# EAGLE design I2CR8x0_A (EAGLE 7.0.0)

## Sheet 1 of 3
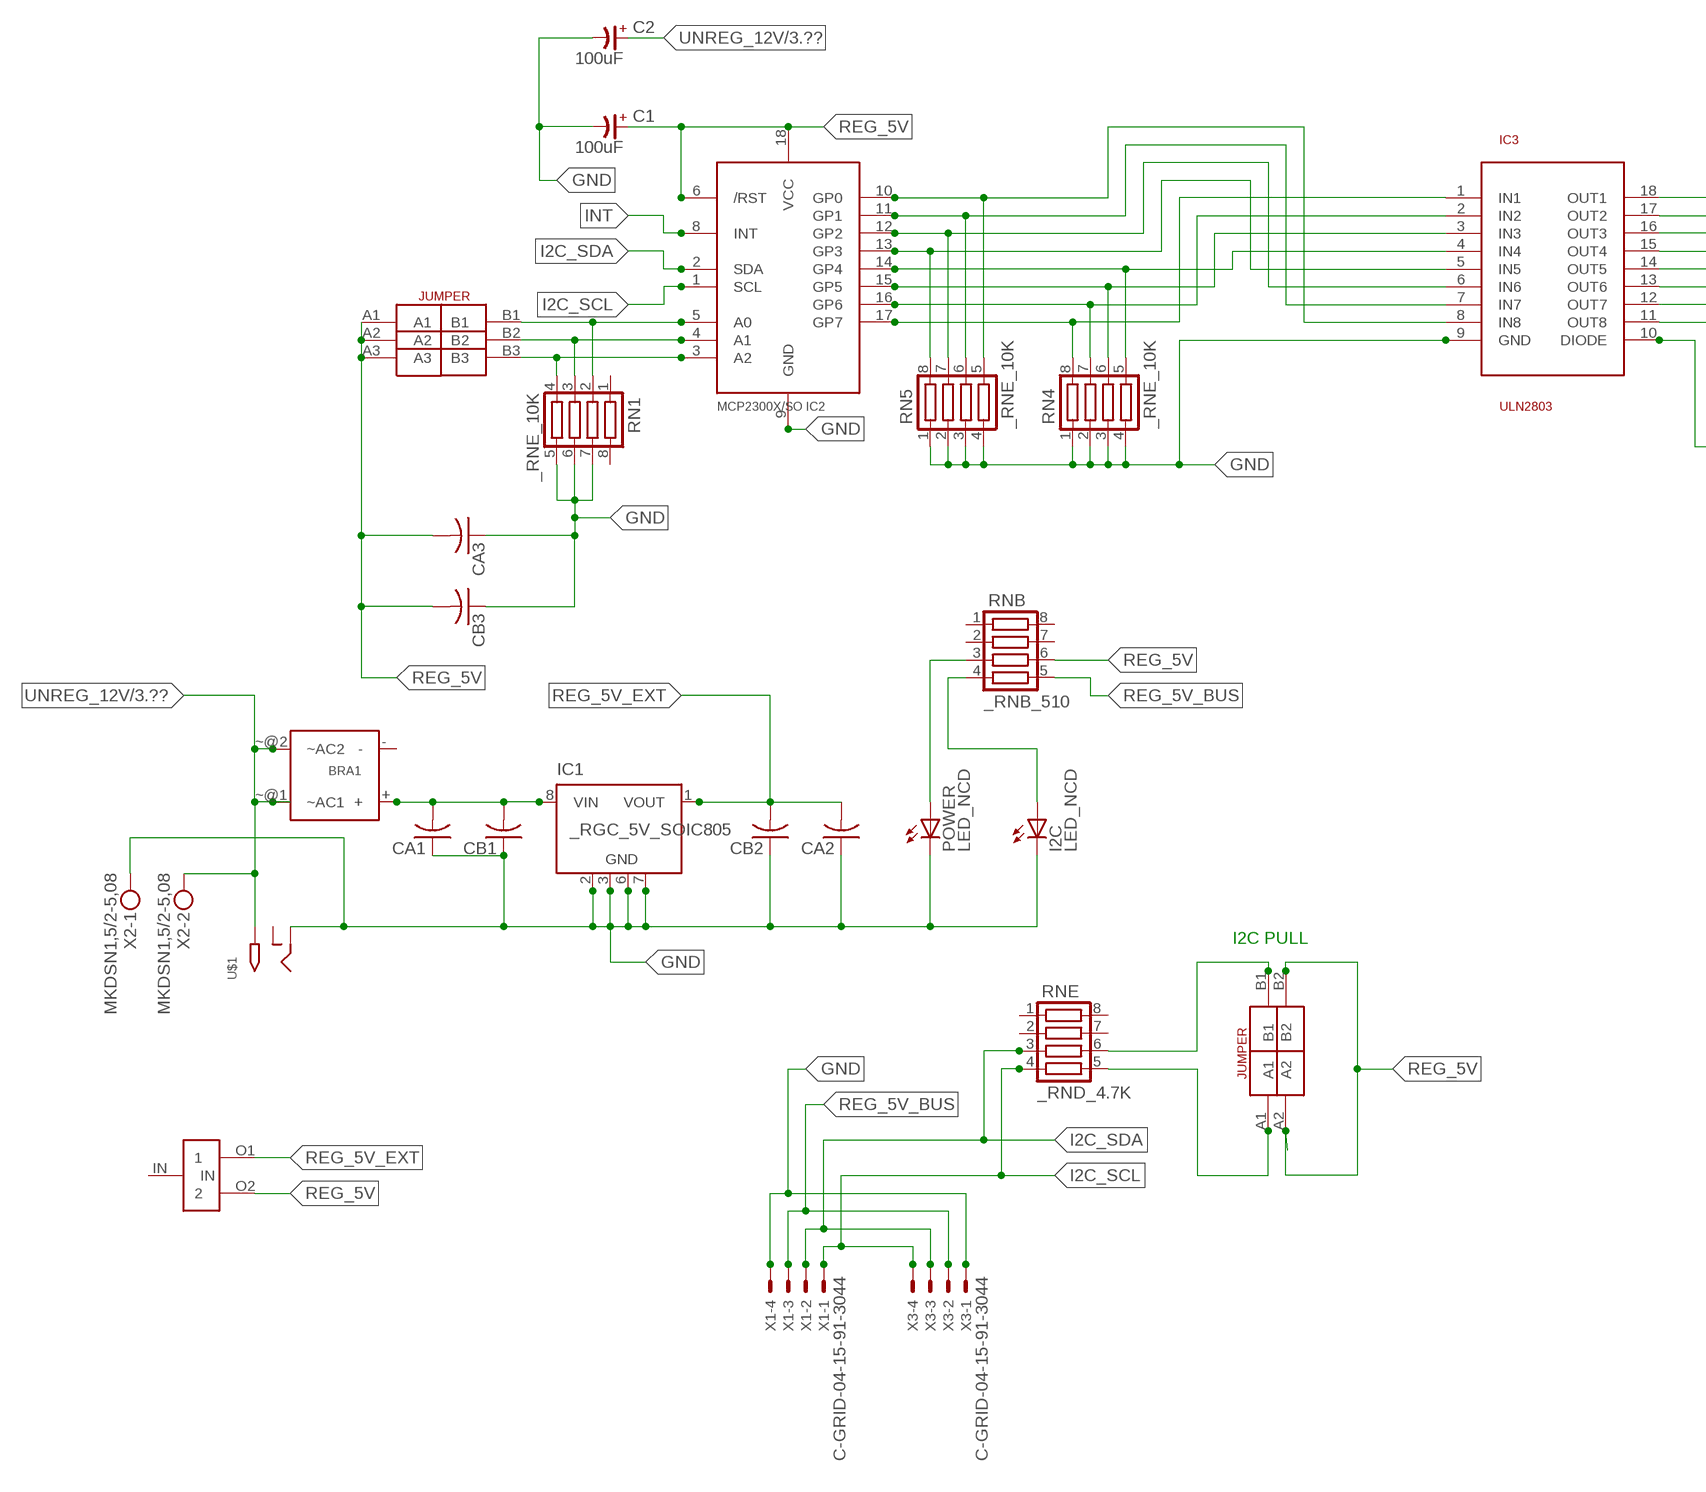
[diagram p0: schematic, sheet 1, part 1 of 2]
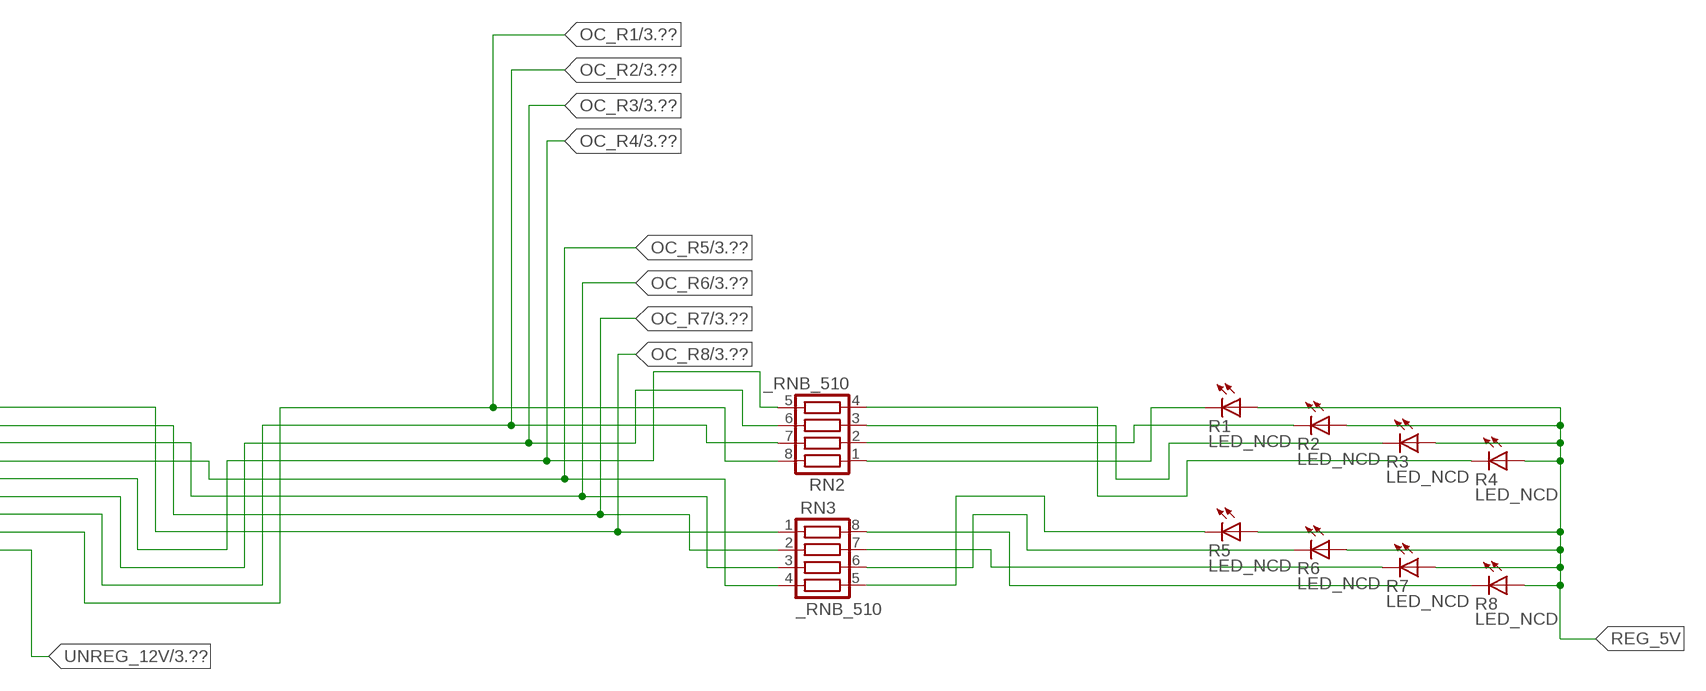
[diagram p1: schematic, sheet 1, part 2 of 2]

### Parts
BRA1  MB2S_  [MB2S]
C1  100uF  CP-E-025X060  [E-025X060]
C2  100uF  CP-E-025X060  [E-025X060]
CA1  CC1206KRX7R9BB104C1206K  [CC1206KRX7R9BB104]
CA2  CC1206KRX7R9BB104C1206K  [CC1206KRX7R9BB104]
CA3  CC1206KRX7R9BB104C1206K  [CC1206KRX7R9BB104]
CB1  TMK316F106ZL-TC1206K  [TMK316F106ZL-T]
CB2  TMK316F106ZL-TC1206K  [TMK316F106ZL-T]
CB3  TMK316F106ZL-TC1206K  [TMK316F106ZL-T]
I2C  LED_NCD  [CHIPLED_0603]
IC1  _RGC_5V_SOIC805  [_RGC_5V_SOIC8]
IC2  MCP2300X/SO  [SO18W]
IC3  ULN2803  [SO18L]
POWER  LED_NCD  [CHIPLED_0603]
R1  LED_NCD  [CHIPLED_0603]
R2  LED_NCD  [CHIPLED_0603]
R3  LED_NCD  [CHIPLED_0603]
R4  LED_NCD  [CHIPLED_0603]
R5  LED_NCD  [CHIPLED_0603]
R6  LED_NCD  [CHIPLED_0603]
R7  LED_NCD  [CHIPLED_0603]
R8  LED_NCD  [CHIPLED_0603]
RN1  _RNE_10K  [RNE]
RN2  _RNB_510  [RNB]
RN3  _RNB_510  [RNB]
RN4  _RNE_10K  [RNE]
RN5  _RNE_10K  [RNE]
RNB  _RNB_510  [RNB]
RNE  _RND_4.7K  [RND]
U$1  2.1MMJACK  [PJ-102A]
U$3  JUMPER_2X2  [JUMPER_2X2]
U$5  LINK_2  [LINK_2]
U$18  JUMPER_3X2  [JUMPER_3X2]
X1  C-GRID-04-15-91-3044  [15-91-04]
X2  MKDSN1,5/2-5,08  [MKDSN1,5/2-5,08]
X3  C-GRID-04-15-91-3044  [15-91-04]

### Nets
GND: C1.- C2.- CA1.1 CA2.1 CA3.1 CB1.1 CB2.1 CB3.1 I2C.C IC1.2(GND) IC1.3(GND) IC1.6(GND) IC1.7(GND) IC2.9(GND) IC3.9(GND) POWER.C RN1.5 RN1.6 RN1.7 RN4.1 RN4.2 RN4.3 RN4.4 RN5.1 RN5.2 RN5.3 RN5.4 U$1.RING X1.4 X2.1 X3.1
GP4: IC2.14(GP4) IC3.4(IN4) RN4.5
GP6: IC2.16(GP6) IC3.2(IN2) RN4.7
I2C_SCL: IC2.1(SCL) RNE.4 X1.1 X3.4
I2C_SDA: IC2.2(SDA) RNE.3 X1.2 X3.3
INT: IC2.8(INT)
N$1: BRA1.+ CA1.2 CB1.2 IC1.8(VIN)
N$2: POWER.A RNB.3
N$3: I2C.A RNB.4
N$4: RNE.5 U$3.A1
N$5: RNE.6 U$3.B1
N$6: IC2.5(A0) RN1.2 U$18.B1
N$7: IC2.4(A1) RN1.3 U$18.B2
N$8: IC2.3(A2) RN1.4 U$18.B3
N$20: R1.C RN2.1
N$21: IC2.12(GP2) IC3.6(IN6) RN5.7
N$22: IC2.11(GP1) IC3.7(IN7) RN5.6
N$23: IC2.10(GP0) IC3.8(IN8) RN5.5
N$29: R2.C RN2.2
N$30: R3.C RN2.3
N$31: R4.C RN2.4
N$32: R8.C RN3.8
N$81: R7.C RN3.7
N$82: R6.C RN3.6
N$83: R5.C RN3.5
N$89: IC2.13(GP3) IC3.5(IN5) RN5.8
N$93: IC2.15(GP5) IC3.3(IN3) RN4.6
N$94: IC2.17(GP7) IC3.1(IN1) RN4.8
OC_R1: IC3.11(OUT8) RN2.8 ; also sheet 3
OC_R2: IC3.12(OUT7) RN2.7 ; also sheet 3
OC_R3: IC3.13(OUT6) RN2.6 ; also sheet 3
OC_R4: IC3.14(OUT5) RN2.5 ; also sheet 3
OC_R5: IC3.15(OUT4) RN3.4 ; also sheet 3
OC_R6: IC3.16(OUT3) RN3.3 ; also sheet 3
OC_R7: IC3.17(OUT2) RN3.2 ; also sheet 3
OC_R8: IC3.18(OUT1) RN3.1 ; also sheet 3
REG_5V: C1.+ CA3.2 CB3.2 IC2.6(/RST) IC2.18(VCC) R1.A R2.A R3.A R4.A R5.A R6.A R7.A R8.A RNB.6 U$3.A2 U$3.B2 U$5.O2 U$18.A1 U$18.A2 U$18.A3
REG_5V_BUS: RNB.5 X1.3 X3.2
REG_5V_EXT: CA2.2 CB2.2 IC1.1(VOUT) U$5.O1
UNREG_12V: BRA1.~@1(~AC1) BRA1.~@2(~AC2) C2.+ IC3.10(DIODE) U$1.TIP X2.2 ; also sheet 3
Unconnected: BRA1.- IC1.4(NC) IC1.5(NC) RN1.1 RN1.8 RNB.1 RNB.2 RNB.7 RNB.8 RNE.1 RNE.2 RNE.7 RNE.8 U$1.RING_SW U$5.IN

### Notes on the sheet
- I2C PULL

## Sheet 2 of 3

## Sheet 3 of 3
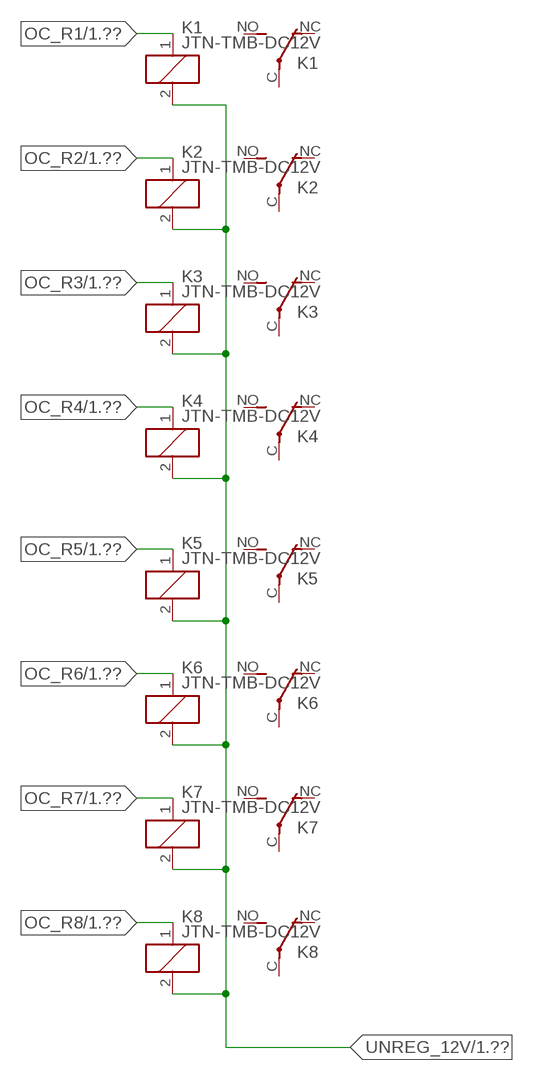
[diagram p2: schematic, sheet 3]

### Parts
K1  JTN-TMB-DC12V  [JT-TMB]
K2  JTN-TMB-DC12V  [JT-TMB]
K3  JTN-TMB-DC12V  [JT-TMB]
K4  JTN-TMB-DC12V  [JT-TMB]
K5  JTN-TMB-DC12V  [JT-TMB]
K6  JTN-TMB-DC12V  [JT-TMB]
K7  JTN-TMB-DC12V  [JT-TMB]
K8  JTN-TMB-DC12V  [JT-TMB]

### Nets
OC_R1: K1.1(C1) ; also sheet 1
OC_R2: K2.1(C1) ; also sheet 1
OC_R3: K3.1(C1) ; also sheet 1
OC_R4: K4.1(C1) ; also sheet 1
OC_R5: K5.1(C1) ; also sheet 1
OC_R6: K6.1(C1) ; also sheet 1
OC_R7: K7.1(C1) ; also sheet 1
OC_R8: K8.1(C1) ; also sheet 1
UNREG_12V: K1.2(C2) K2.2(C2) K3.2(C2) K4.2(C2) K5.2(C2) K6.2(C2) K7.2(C2) K8.2(C2) ; also sheet 1
Unconnected: K1.C(COM) K1.NC K1.NO K2.C(COM) K2.NC K2.NO K3.C(COM) K3.NC K3.NO K4.C(COM) K4.NC K4.NO K5.C(COM) K5.NC K5.NO K6.C(COM) K6.NC K6.NO K7.C(COM) K7.NC K7.NO K8.C(COM) K8.NC K8.NO

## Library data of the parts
BRA1 = NCD_ULTIMATE_LIBRARY:MB2S: Bridge Rectifier BRA MB2S 200V 500ma Digikey MB2S-TPMSTR-ND/MB2S-TP
C1 C2 = NCD_ULTIMATE_LIBRARY:CP-: Capacitors All Kinds POLARIZED CAP
CA1-CA3 = NCD_ULTIMATE_LIBRARY:CC1206KRX7R9BB104: Capacitor CA .1uF 50V SMT C1206K CC1206KRX7R9BB104
CB1-CB3 = NCD_ULTIMATE_LIBRARY:TMK316F106ZL-T: Capacitor CB 10uF SMT 1206 TMK316F106ZL-T
I2C POWER = NCD_ULTIMATE_bhaskar:LED_NCD
IC1 = NCD_ULTIMATE_LIBRARY:_RGC_5V_SOIC8: Regulator Linear 5V Chip Positive VOLTAGE REGULATOR Digikey 497-7267-2-ND/L78L05CD13TR
IC2 = NCD_ULTIMATE_LIBRARY:MCP2300X: Semiconductor Port Expander I/O 8-Bit I2C MCP23008 Inexpensive i2c i/o expander - 8 general purpose i/o pins with optional pullups
IC3 = NCD_ULTIMATE_LIBRARY:ULN2803: Semiconductor 8 O.C. N-Channel Transistor Driver Digikey ULN2803AFWGCELTR-ND/ULN2803AFWG,C,EL
K1-K8 = NCD_ULTIMATE_LIBRARY:JT?-*: RELAY COMPACT ECONOMICAL 30 AMP. RELAY NAiS Source: http://www.mew-europe.com/.. en_ds_61212_0000.pdf
R1-R8 = NCD_ULTIMATE_LIBRARY:LED_NCD: LED Digikey 754-1132-2-ND/APT2012SRCPRV
RN1 RN4 RN5 = NCD_ULTIMATE_LIBRARY:_RNE_10K: Resistor Array RNE SMT 10K x 4 Single Resistor Source: http://www.ctscorp.com/components/Datasheets/CTSChipArrayDs.pdf Digikey 742C083103JPTR-ND/742C083103JP; OC_FARNELL: unknown; OC_NEWARK: unknown
RN2 RN3 RNB = NCD_ULTIMATE_LIBRARY:_RNB_510: Resistor Array RNB SMT 510 x 4 Single Resistor Source: http://www.ctscorp.com/components/Datasheets/CTSChipArrayDs.pdf Digikey 742C083511JPTR-ND/ 742C083511JP; OC_FARNELL: unknown; OC_NEWARK: unknown
RNE = NCD_ULTIMATE_LIBRARY:_RND_4.7K: Resistor Array RND SMT 4.7K x 4 Single Resistor Source: http://www.ctscorp.com/components/Datasheets/CTSChipArrayDs.pdf Digikey 742C083472JPTR-ND/742C083472JP; OC_FARNELL: unknown; OC_NEWARK: unknown
U$1 = NCD_ULTIMATE_CONNECTORS:2.1MMJACK: 2.1mm x 5.5mm DC jack with internal switch. Digikey part #PJ-102A, 4UCON part #05537 By microbuilder.eu
U$3 = NCD_ULTIMATE_CONNECTORS:JUMPER_2X2
U$5 = NCD_ULTIMATE_LIBRARY:LINK_2: PAD_top
U$18 = NCD_ULTIMATE_CONNECTORS:JUMPER_3X2
X1 X3 = NCD_ULTIMATE_CONNECTORS:C-GRID-04: CONNECTOR 4-Pos I2C wire to board 2.54 mm (0.100") pitch header Digikey WM1342-ND/0015912045; OC_FARNELL: unknown; OC_NEWARK: unknown
X2 = NCD_ULTIMATE_CONNECTORS:MKDSN1,5/2-5,08: MKDSN 1,5/ 2-5,08 Printklemme

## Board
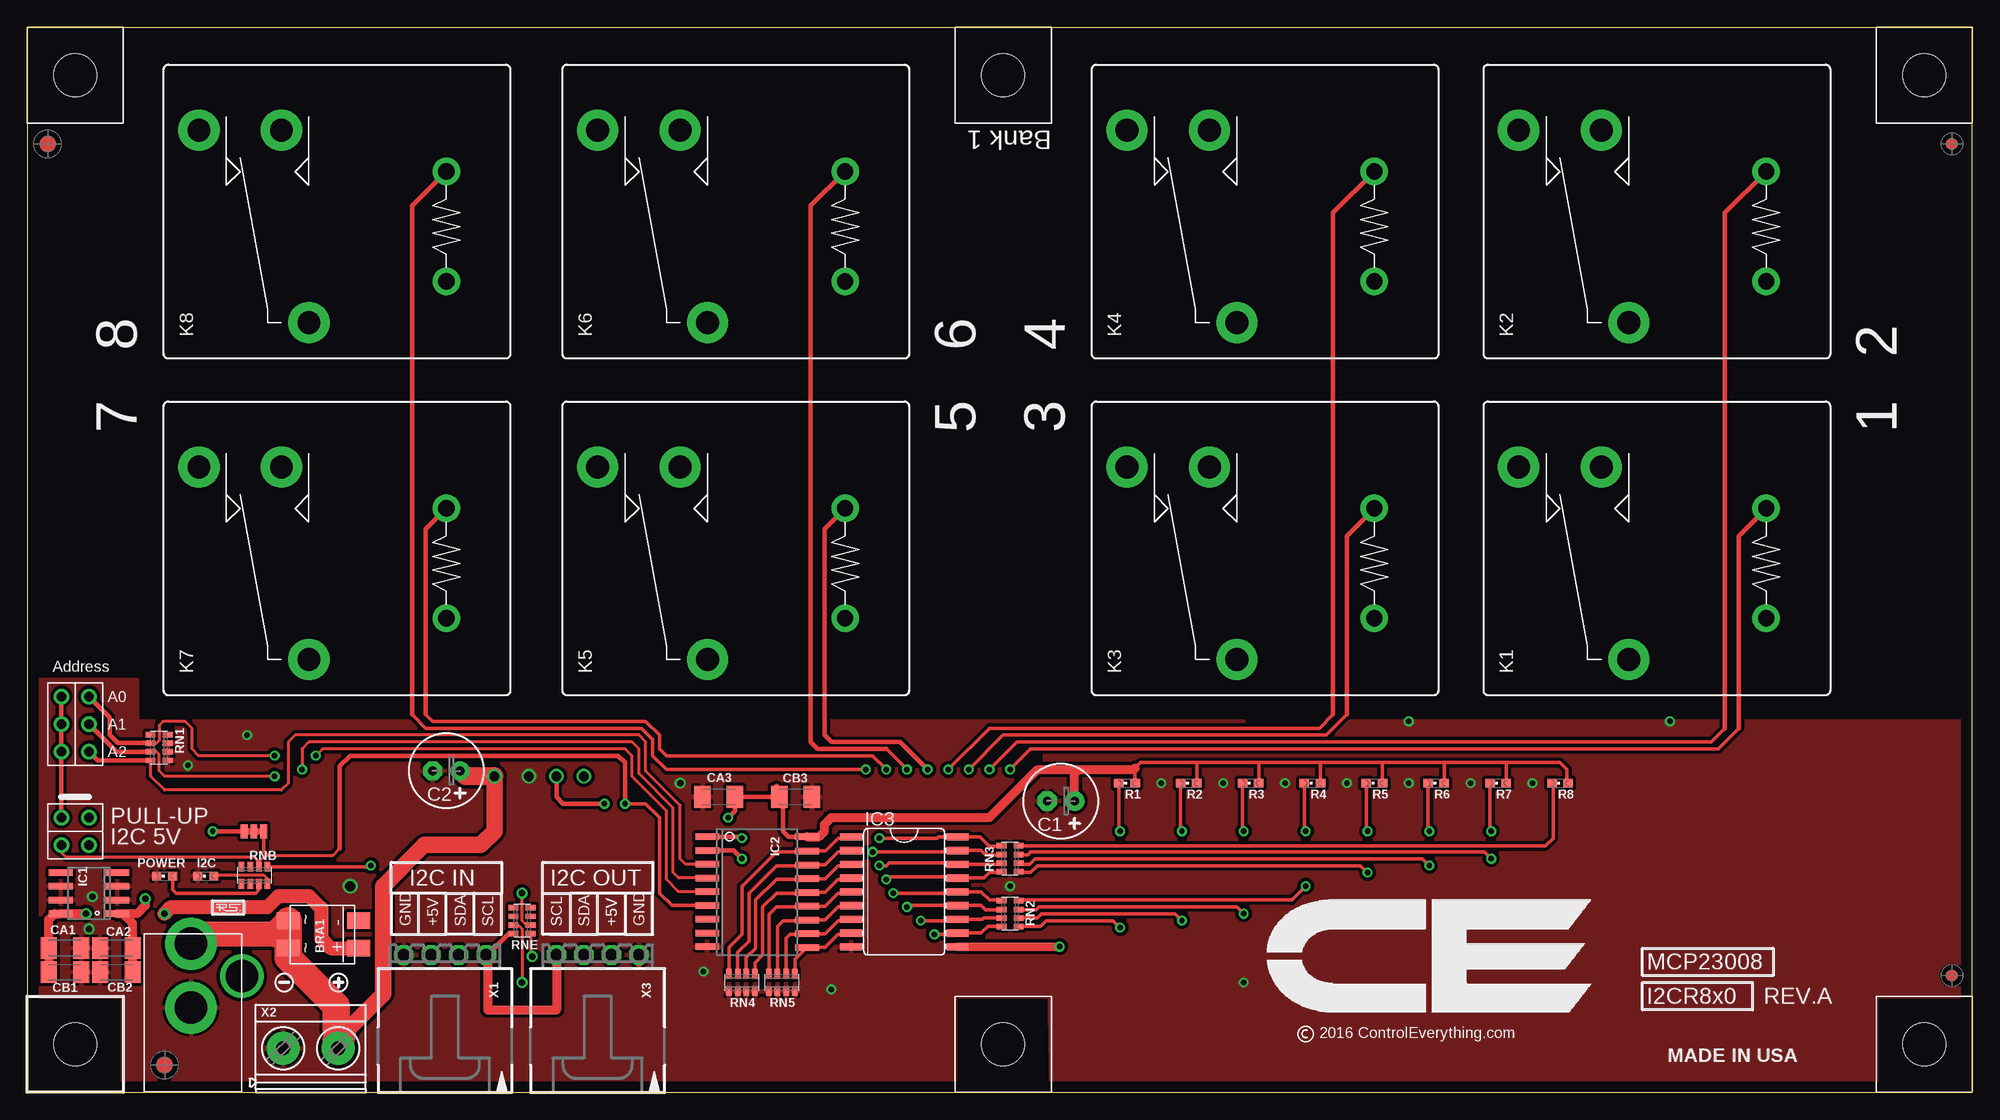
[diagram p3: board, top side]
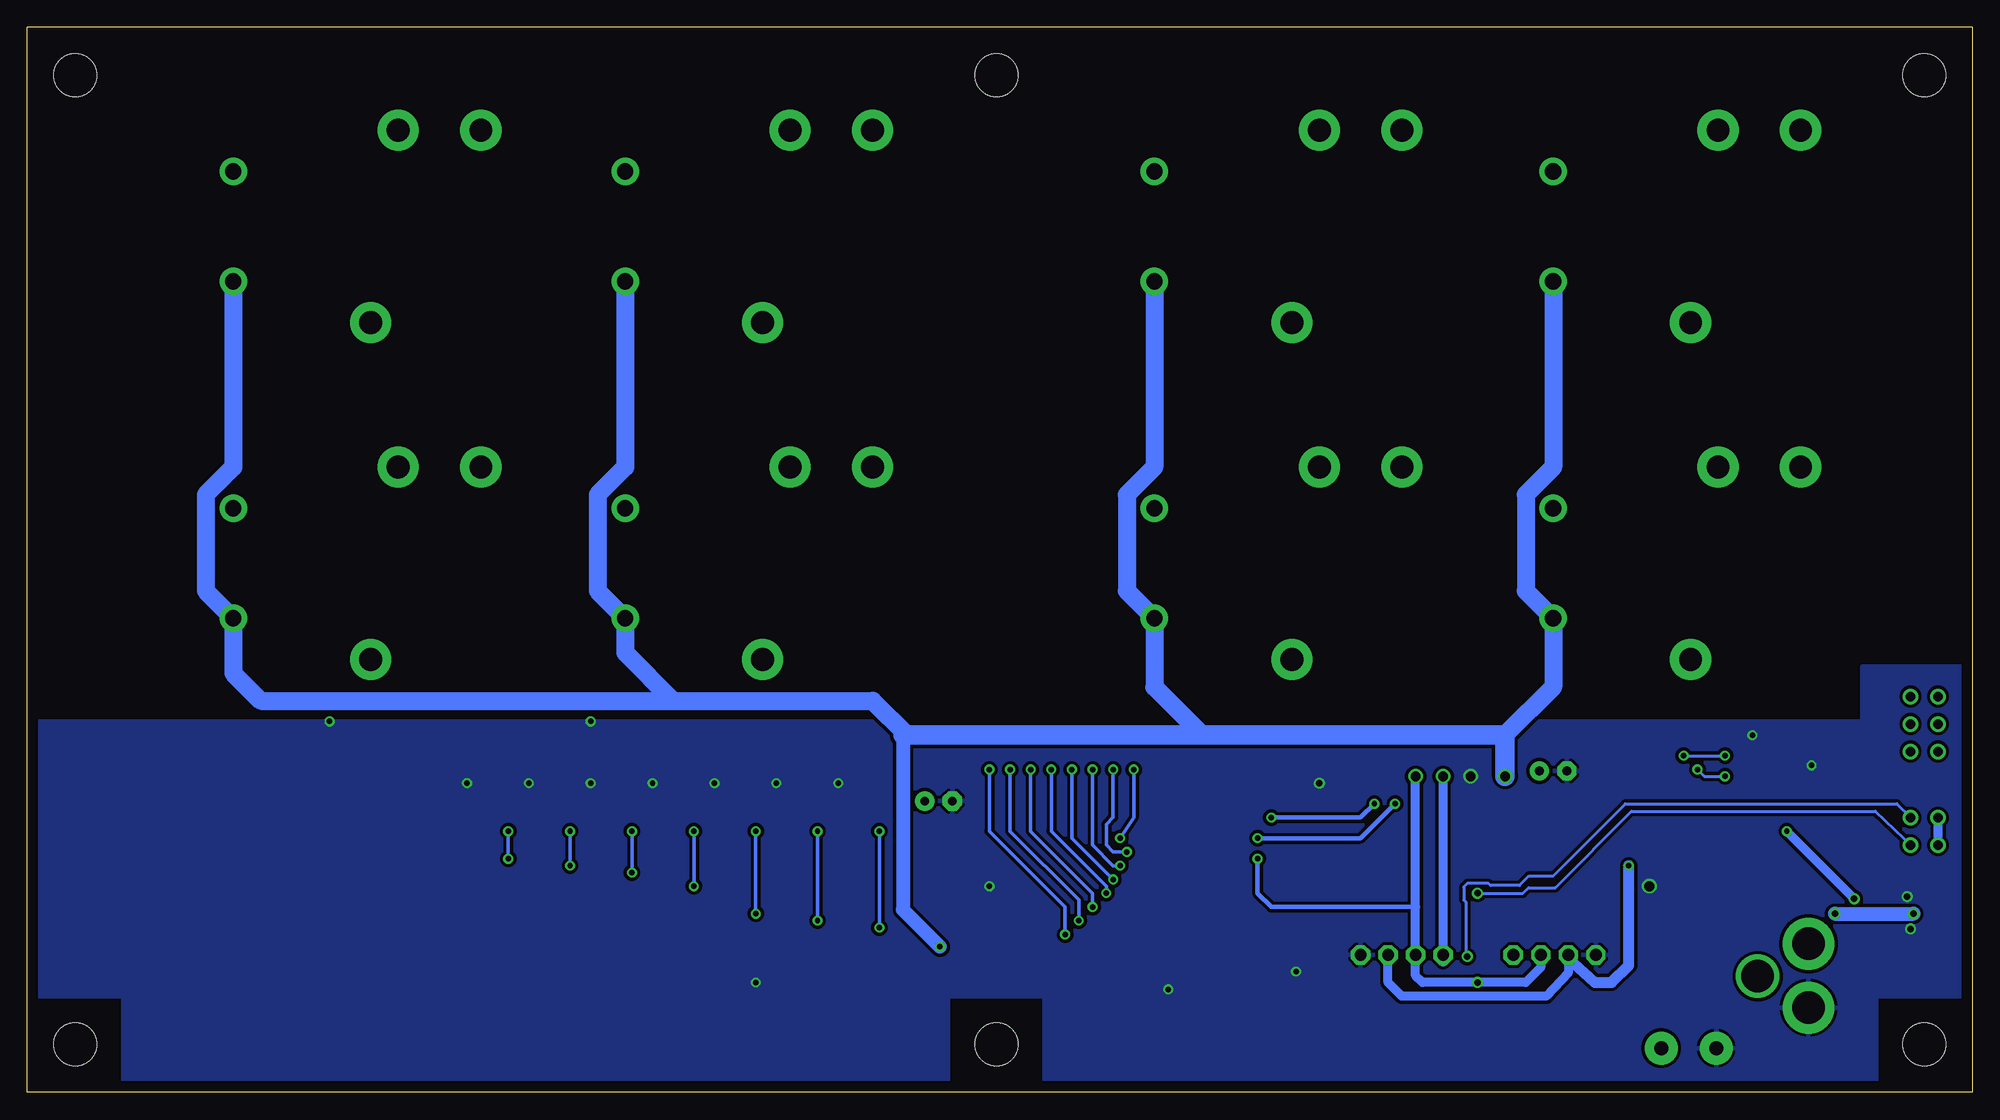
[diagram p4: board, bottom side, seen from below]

Size 179.71 x 98.44 mm. Coordinates in mm from the lower left corner, seen from the top.
Outline: 81.28,0 0,0 0,55.88
Outline: 81.28,0 82.53,0
Outline: 0,56.82 0,55.88
Outline: 81.28,0 179.71,0 179.71,98.42
Outline: 0,98.42 0,55.88
Outline: 0.02,98.44 179.71,98.44
Copper layers (1*16): Top 0.035mm / dielectric 1.5mm / Bottom 0.035mm
Design rules "default": minimum track width 10mil, minimum drill 24mil, track to track 8mil, track to pad 8mil, pad to pad 8mil, via to via 8mil, smd to smd 8mil, copper to edge 40mil, drill to drill 8mil, minimum pad ring 10mil, minimum via ring 8mil, stop-mask expansion 4mil, vias tented up to drill 0mil, thermal gap 10mil
Holes 3.96 mm at 4.45,4.45

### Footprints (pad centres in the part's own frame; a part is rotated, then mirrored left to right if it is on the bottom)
MB2S = smd 1.55 x 2.1: + 0,-6.5; - 2.54,-6.5; ~@1 0,0; ~@2 2.54,0
E-025X060 = drill 0.813 pad 1.778: + -1.27,0 | drill 0.813 pad 1.778 octagon: - 1.27,0
CC1206KRX7R9BB104 = smd 1.5 x 2: 1 -1.5,0; 2 1.5,0
TMK316F106ZL-T = smd 1.5 x 2: 1 -1.5,0; 2 1.5,0
CHIPLED_0603 = smd 0.8 x 0.8: A 0,-0.75; C 0,0.75
_RGC_5V_SOIC8 = smd 0.6 x 2.2: 1 -1.905,-2.6; 2 -0.635,-2.6; 3 0.635,-2.6; 4 1.905,-2.6; 5 1.905,2.6; 6 0.635,2.6; 7 -0.635,2.6; 8 -1.905,2.6
SO18W = smd 0.6 x 2.2: 1 -4.445,-4.6; 2 -3.175,-4.6; 3 -1.905,-4.6; 4 -0.635,-4.6; 5 0.635,-4.6; 6 1.905,-4.6; 7 3.175,-4.6; 8 4.445,-4.6; 9 5.715,-4.6; 10 5.775,4.6; 11 4.505,4.6; 12 3.235,4.6; 13 1.965,4.6; 14 0.695,4.6; 15 -0.575,4.6; 16 -1.845,4.6; 17 -3.145,4.6; 18 -4.445,4.6
SO18L = smd 0.66 x 2.032: 1 -5.08,-4.902; 2 -3.81,-4.902; 3 -2.54,-4.902; 4 -1.27,-4.902; 5 0,-4.902; 6 1.27,-4.902; 7 2.54,-4.902; 8 3.81,-4.902; 9 5.08,-4.902; 10 5.08,4.902; 11 3.81,4.902; 12 2.54,4.902; 13 1.27,4.902; 14 0,4.902; 15 -1.27,4.902; 16 -2.54,4.902; 17 -3.81,4.902; 18 -5.08,4.902
JT-TMB = drill 1.5 pad 2.54: 1 5.08,0; 2 -5.08,0 | drill 2.1 pad 3.81: C -8.89,12.7; NC 8.89,22.86; NO 8.89,15.24
CHIPLED_0603' = smd 0.8 x 0.876: A 0,-0.75; C 0,0.75
RNE = smd 0.5 x 0.9: 1 -1.2,-0.8; 2 -0.4,-0.8; 3 0.4,-0.8; 4 1.2,-0.8; 5 1.2,0.8; 6 0.4,0.8; 7 -0.4,0.8; 8 -1.2,0.8
RNB = smd 0.5 x 0.9: 1 -1.2,-0.8; 2 -0.4,-0.8; 3 0.4,-0.8; 4 1.2,-0.8; 5 1.2,0.8; 6 0.4,0.8; 7 -0.4,0.8; 8 -1.2,0.8
RND = smd 0.5 x 0.9: 1 -1.2,-0.8; 2 -0.4,-0.8; 3 0.4,-0.8; 4 1.2,-0.8; 5 1.2,0.8; 6 0.4,0.8; 7 -0.4,0.8; 8 -1.2,0.8
PJ-102A = drill 3 pad 4.8: RING 0.1,-3.39; TIP 0.1,-9.29 | drill 3 pad 3.251: RING_SW -4.6,-6.29
JUMPER_2X2 = drill 0.9: A1 0,2.54; A2 0,0; B1 2.54,2.54; B2 2.54,0
LINK_2 = smd 1.27 x 0.635: IN 0,0; O1 0,0.889; O2 0,-0.889
PCB_MOUNTING_HOLE = hole 3.962: 4.445,4.445
JUMPER_3X2 = drill 0.9: A1 0,5.08; A2 0,2.54; A3 0,0; B1 2.54,5.08; B2 2.54,2.54; B3 2.54,0
15-91-04 = drill 1.1 pad 1.778 octagon: 1 -3.81,-7.62; 2 -1.27,-7.62; 3 1.27,-7.62; 4 3.81,-7.62
MKDSN1,5/2-5,08 = drill 1.3 pad 3.048: 1 -2.561,0.025; 2 2.519,0.025

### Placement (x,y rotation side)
BRA1  24.13,13.34 90 top
C1  95.5,26.92 180 top
C2  38.73,29.72 180 top
CA1  3.49,13.34 180 top
CA2  8.26,13.34 0 top
CA3  63.88,27.3 0 top
CB1  3.49,11.11 180 top
CB2  8.26,11.11 0 top
CB3  70.99,27.3 180 top
I2C  16.51,20 90 top
IC1  5.71,18.41 90 top
IC2  67.44,19.18 270 top
IC3  81.03,18.54 270 top
K1  160.66,48.9 90 top
K2  160.66,80.01 90 top
K3  124.46,48.9 90 top
K4  124.46,80.01 90 top
K5  75.56,48.9 90 top
K6  75.56,80.01 90 top
K7  38.73,48.9 90 top
K8  38.73,80.01 90 top
POWER  12.7,20 90 top
R1  LED_NCD  [CHIPLED_0603']  101.6,28.57 90 top
R2  LED_NCD  [CHIPLED_0603']  107.31,28.57 90 top
R3  LED_NCD  [CHIPLED_0603']  113.03,28.57 90 top
R4  LED_NCD  [CHIPLED_0603']  118.75,28.57 90 top
R5  LED_NCD  [CHIPLED_0603']  124.46,28.57 90 top
R6  LED_NCD  [CHIPLED_0603']  130.18,28.57 90 top
R7  LED_NCD  [CHIPLED_0603']  135.89,28.57 90 top
R8  LED_NCD  [CHIPLED_0603']  141.6,28.57 90 top
RN1  12.19,31.88 270 top
RN2  90.81,16.51 90 top
RN3  90.81,21.59 270 top
RN4  66.04,10.16 0 top
RN5  69.72,10.16 0 top
RNB  21.02,20.07 0 top
RNE  45.72,15.88 270 top
U$1  15.24,4.45 180 top
U$3  3.17,25.4 270 top
U$4  [VISION_REF10]  177.8,10.79 270 top
U$5  20.95,24.13 90 top
U$6  PCB_MOUNTING_HOLE  [PCB_MOUNTING_HOLE]  94.61,0 90 top
U$10  [VISION_REF15]  12.7,2.54 0 top
U$11  PCB_MOUNTING_HOLE  [PCB_MOUNTING_HOLE]  179.71,0 90 top
U$13  [VISION_REF10]  177.8,87.63 270 top
U$14  [VISION_REF15]  1.91,87.63 270 top
U$17  PCB_MOUNTING_HOLE  [PCB_MOUNTING_HOLE]  94.61,89.53 90 top
U$18  3.17,31.5 0 top
U$19  PCB_MOUNTING_HOLE  [PCB_MOUNTING_HOLE]  94.61,89.53 90 top
U$20  PCB_MOUNTING_HOLE  [PCB_MOUNTING_HOLE]  179.71,89.53 90 top
U$21  [ICON_USA]  151.51,2.79 0 top
U$22  [ICON_MINUS]  23.75,10.16 180 top
U$24  [ICON_PLUS]  28.77,10.16 90 top
U$25  PCB_MOUNTING_HOLE  [PCB_MOUNTING_HOLE]  179.71,89.53 90 top
U$31  PCB_MOUNTING_HOLE  [PCB_MOUNTING_HOLE]  8.89,89.53 90 top
U$32  PCB_MOUNTING_HOLE  [PCB_MOUNTING_HOLE]  8.89,89.53 90 top
X1  38.61,5.08 180 top
X2  26.23,4.06 0 top
X3  52.7,5.08 180 top

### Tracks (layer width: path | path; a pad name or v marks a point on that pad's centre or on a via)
GND  (via drill 0.5, 0.6, 0.9)
  Top 0.406: 34.8,12.38 X1.4
  Top 0.813: X3.1 56.52,12.06
  other vias: 5.71,15.11 6.03,18.1 46.35,29.21 29.84,19.05 14.86,30.23 62.48,11.18 127.64,28.57 112.39,10.16 133.35,28.57 139.06,28.57 121.92,28.57 116.2,28.57 110.49,28.57 104.78,28.57 90.81,19.05 127.64,34.29 151.76,34.29 74.3,9.53 20.32,33.02 60.33,28.57
  pour Bottom (isolate 0.305): 0.64,8.89 8.89,8.89 8.89,0 85.72,0 85.72,8.89 112.39,8.89 112.39,34.29 10.16,34.29 10.16,39.37 0.64,39.37
  pour Top (isolate 0.305): 0.64,8.89 8.89,8.89 8.89,0 85.72,0 85.72,8.89 112.39,8.89 112.39,34.29 10.16,34.29 10.16,38.1 -1.27,38.1
  pour Top (isolate 0.305): 112.39,34.29 179.07,34.29 179.07,8.89 170.81,8.89 170.81,0 112.39,0
  pour Bottom (isolate 0.305): 94.61,0 94.61,34.29 179.07,34.29 179.07,8.89 170.81,8.89 170.81,0
  pour Top (isolate 0.305): 179.07,8.89 170.81,8.89 170.81,0 94.61,0 95.25,34.29 179.07,34.29
  pour Top (isolate 0.305): 170.81,8.89 170.81,0 94.61,0 93.98,34.29 179.07,34.29 179.07,8.89
GP4
  Top 0.305: RN4.5 67.24,11.99 67.94,12.7 67.94,17.14 69.22,18.41 71.97,18.41 IC2.14 73.73,18.48 74.93,19.68 76,19.68 IC3.4
GP6
  Top 0.305: RN4.7 65.64,12.94 66.67,13.97 66.67,18.41 69.22,20.95 71.97,20.95 IC2.16 73.73,21.02 74.93,22.23 76,22.23 IC3.2
I2C_SCL  (via drill 0.5, 0.9)
  Top 0.406: RNE.4 44.51,14.68 42.55,12.7 | IC2.1 65.91,23.62 v66.04,23.5 | v53.34,26.67 49.53,26.67 48.9,27.3 v48.9,29.21
  Top 0.813: X3.4 48.9,7.62 42.55,7.62 42.55,12.7 X1.1
  Bottom 0.406: v66.04,23.5 56.52,23.5 v53.34,26.67
  Bottom 0.813: v48.9,29.21 X3.4 48.9,12.06
I2C_SDA  (via drill 0.5, 0.6, 0.9)
  Top 0.254: RNE.3 45.36,15.47 45.72,15.11 v45.72,10.16
  Top 0.406: IC2.2 65.28,22.35 v66.04,21.59
  Top 0.61: X3.3 51.44,12.06 | X1.2 39.88,12.38
  Bottom 0.406: v66.04,21.59 66.04,18.41 64.77,17.14 51.44,17.14 | 39.88,12.38 X1.2
  Bottom 0.813: 39.88,12.38 39.88,11.56 41.27,10.16 v45.72,10.16 50.8,10.16 51.44,10.79 X3.3 51.44,17.14 v51.44,29.21
N$1  (via drill 0.6)
  Top 0.813: CB1.2 CA1.2 1.99,15.96 2.54,16.51 IC1.8 v5.46,16.51
  Top 1.27: v12.7,16.51 13.34,17.14 22.23,17.14 23.24,18.16 26.04,18.16 27.18,17.02 27.18,14.22 28.07,13.34 BRA1.+
  Bottom 1.27: v12.7,16.51 v5.46,16.51
N$2
  Top 0.305: RNB.3 21.4,18.95 21.4,18.7 21.12,18.41 13.78,18.41 13.45,18.74 POWER.A
N$3
  Top 0.254: 22.23,18.95 22.23,19.74 21.9,20.07 16.94,20.07
  Top 0.305: RNB.4 22.23,18.95 | 16.94,20.07 I2C.A
N$4  (via drill 0.6)
  Top 0.254: RNE.5 46.52,12.6 v46.67,12.57
  Bottom 0.254: U$3.A1 6.99,26.67 32.07,26.67 38.73,20 40.96,20 41.85,19.11 44.51,19.11 44.7,19.3 46.67,19.3 46.99,18.99 46.99,17.78 46.8,17.59 46.8,12.7 v46.67,12.57
N$5  (via drill 0.6)
  Top 0.254: RNE.6 46.12,15.47 45.72,15.88 v45.72,18.41
  Bottom 0.254: v45.72,18.41 41.53,18.41 41.02,18.92 38.54,18.92 31.5,25.97 8.95,25.97 6.35,23.5 U$3.B1
N$6  (via drill 0.5)
  Top 0.254: IC2.5 60.2,18.54 59.05,19.68 59.05,26.04 55.88,29.21 55.88,31.11 55.24,31.75 27.3,31.75 v26.67,31.11 | v22.86,31.11 15.88,31.11 15.24,31.75 15.24,33.66 14.61,34.29 12.57,34.29 12.19,33.91 12.19,32.51 11.94,32.26 11.41,32.26 RN1.2
  Top 0.406: RN1.2 8.36,32.28 7.62,33.02 7.62,34.67 U$18.B1
  Bottom 0.254: v26.67,31.11 v22.86,31.11
N$7  (via drill 0.5)
  Top 0.254: IC2.4 60.2,19.81 59.69,20.32 59.69,26.29 56.52,29.46 56.52,31.75 55.88,32.38 26.04,32.38 25.4,31.75 v25.4,29.84 | v22.86,29.21 12.7,29.21 12.19,29.72 12.19,31.24 11.94,31.5 11.41,31.5 RN1.3
  Top 0.406: RN1.3 8.27,31.48 U$18.B2
  Bottom 0.254: v25.4,29.84 24.77,29.21 v22.86,29.21
N$8
  Top 0.254: IC2.3 60.83,21.08 60.33,21.59 60.33,26.54 57.15,29.72 57.15,32.38 56.52,33.02 24.77,33.02 24.13,32.38 24.13,28.57 23.5,27.94 12.7,27.94 11.43,29.21 11.43,30.64 RN1.4
  Top 0.406: RN1.4 6.53,30.68 U$18.B3
N$20  (via drill 0.5)
  Top 0.305: R1.C 100.85,24.25 v100.97,24.13 | v100.97,15.24 100.33,15.88 94.11,15.88 93.6,15.37 91.66,15.37 RN2.1
  Bottom 0.305: v100.97,24.13 v100.97,15.24
N$21
  Top 0.305: RN5.7 69.32,15.35 69.85,15.88 71.97,15.88 IC2.12 73.73,15.94 74.93,17.14 76,17.14 IC3.6
N$22
  Top 0.305: RN5.6 70.12,14.24 70.48,14.61 71.97,14.61 IC2.11 73.73,14.67 74.93,15.88 76,15.88 IC3.7
N$23
  Top 0.254: 71.97,13.34 IC2.10
  Top 0.305: RN5.5 70.92,12.29 IC2.10 73.73,13.4 74.93,14.61 76,14.61 IC3.8
N$29  (via drill 0.5)
  Top 0.305: R2.C 106.56,24.25 v106.68,24.13 | v106.68,15.88 106.05,16.51 93.73,16.51 93.34,16.13 91.62,16.13 RN2.2
  Bottom 0.305: v106.68,24.13 v106.68,15.88
N$30  (via drill 0.5)
  Top 0.305: R3.C 112.28,24.25 v112.39,24.13 | v112.39,16.51 111.76,17.14 93.47,17.14 93.22,16.89 91.62,16.89 RN2.3
  Bottom 0.305: v112.39,24.13 v112.39,16.51
N$31  (via drill 0.5)
  Top 0.305: R4.C 118,24.25 v118.11,24.13 | v118.11,19.05 116.84,17.78 91.67,17.78 RN2.4
  Bottom 0.305: v118.11,24.13 v118.11,19.05
N$32
  Top 0.305: RN3.8 140.26,22.79 140.97,23.5 140.97,28.46 R8.C
N$81  (via drill 0.5)
  Top 0.305: R7.C 135.14,24.25 v135.25,24.13 | v135.25,21.59 134.62,22.23 92.71,22.23 92.46,21.97 91.62,21.97 RN3.7
  Bottom 0.305: v135.25,24.13 v135.25,21.59
N$82  (via drill 0.5)
  Top 0.305: R6.C 129.43,24.25 v129.54,24.13 | v129.54,20.95 128.91,21.59 93.09,21.59 92.58,21.08 91.71,21.08 RN3.6
  Bottom 0.305: v129.54,24.13 v129.54,20.95
N$83  (via drill 0.5)
  Top 0.305: R5.C 123.71,24.25 v123.83,24.13 | v123.83,20.32 123.19,20.95 93.34,20.95 92.71,20.32 91.67,20.32 RN3.5
  Bottom 0.305: v123.83,24.13 v123.83,20.32
N$89
  Top 0.305: RN5.8 68.52,16.45 69.22,17.14 71.97,17.14 IC2.13 73.73,17.21 74.93,18.41 76,18.41 IC3.5
N$93
  Top 0.305: RN4.6 66.44,12.46 67.31,13.34 67.31,17.78 69.22,19.68 71.97,19.68 IC2.15 73.73,19.75 74.93,20.95 76,20.95 IC3.3
N$94
  Top 0.305: RN4.8 64.84,13.4 66.04,14.61 66.04,19.05 69.22,22.23 71.94,22.23 IC2.17 73.76,22.32 74.93,23.5 76,23.5 IC3.1
OC_R1  (via drill 0.5)
  Top 0.305: RN2.8 89.95,15.37 88.77,15.37 88.14,14.73 IC3.11 85.8,14.61 v83.82,14.61 | v90.81,29.84 92.71,31.75 156.21,31.75 158.12,33.66
  Top 0.406: K1.1 158.12,51.44 158.12,33.66
  Bottom 0.305: v90.81,29.84 90.81,24.13 83.82,17.14 v83.82,14.61
OC_R2  (via drill 0.5)
  Top 0.305: RN2.7 89.99,16.13 88.39,16.13 88.27,16 IC3.12 85.8,15.88 v82.55,15.88 | v88.9,29.84 91.44,32.38 155.57,32.38 156.84,33.66
  Top 0.406: K2.1 156.84,81.28 156.84,33.66
  Bottom 0.305: v88.9,29.84 88.9,24.13 82.55,17.78 v82.55,15.88
OC_R3  (via drill 0.5)
  Top 0.305: RN2.6 89.99,16.89 88.52,16.89 88.14,17.27 IC3.13 81.53,17.27 81.41,17.14 v81.28,17.14 | 121.92,34.92 120.02,33.02 90.17,33.02 v87,29.84
  Top 0.406: K3.1 121.92,51.44 121.92,34.92
  Bottom 0.305: v87,29.84 87,24.13 81.28,18.41 v81.28,17.14
OC_R4  (via drill 0.5)
  Top 0.305: RN2.5 89.94,17.78 88.9,17.78 88.14,18.54 IC3.14 85.8,18.41 v80.01,18.41 | 120.65,34.92 119.38,33.66 88.9,33.66 v85.09,29.84
  Top 0.406: K4.1 120.65,81.28 120.65,34.92
  Bottom 0.305: v85.09,29.84 85.09,24.13 80.01,19.05 v80.01,18.41
OC_R5  (via drill 0.5)
  Top 0.305: RN3.4 89.94,20.32 88.9,20.32 88.39,19.81 IC3.15 85.8,19.94 79.63,19.94 v79.38,19.68
  Top 0.406: K5.1 73.66,52.07 73.66,33.02 74.3,32.38 80.64,32.38 v83.19,29.84
  Bottom 0.305: v83.19,29.84 83.19,23.5 v79.38,19.68
OC_R6  (via drill 0.5)
  Top 0.305: RN3.3 89.9,21.08 IC3.16 85.8,21.21 79.63,21.21 79.38,20.95 v78.74,20.95 | 79.38,31.75 v81.28,29.84
  Top 0.406: K6.1 72.39,81.92 72.39,32.38 73.03,31.75 79.38,31.75
  Bottom 0.305: v81.28,29.84 81.28,22.86 79.38,20.95 v78.74,20.95
OC_R7  (via drill 0.5)
  Top 0.305: RN3.2 89.99,21.97 88.52,21.97 88.14,22.35 IC3.17 85.8,22.23 v78.11,22.23 | v79.38,29.84 78.11,31.11 59.05,31.11 58.42,31.75 58.42,33.02 57.15,34.29 37.47,34.29 36.83,34.92
  Top 0.406: K7.1 36.83,52.07 36.83,34.92
  Bottom 0.305: v79.38,29.84 79.38,25.4 80.01,24.77 80.01,22.86 79.38,22.23 v78.11,22.23
OC_R8  (via drill 0.5)
  Top 0.305: RN3.1 89.95,22.73 88.9,22.73 88.01,23.62 IC3.18 84.2,23.62 84.07,23.5 v78.74,23.5 | v77.47,29.84 59.05,29.84 57.78,31.11 57.78,32.64 56.77,33.66 36.83,33.66 35.56,34.92
  Top 0.406: K8.1 35.56,81.92 35.56,34.92
  Bottom 0.305: v77.47,29.84 77.47,25.4 v78.74,23.5
REG_5V  (via drill 0.5)
  Top 0.254: RNB.6 21.42,21.29 | 21.42,21.29 22.04,21.91 22.23,21.91 28.26,21.91 28.89,22.54 | 21.42,21.29 20.99,21.72 3.62,21.72 3.17,22.16 U$3.B2
  Top 0.305: v55.24,26.67 57.15,26.67 58.42,25.4 58.42,18.41 59.56,17.27 IC2.6 | R1.A 102.35,29.96 102.87,30.48 107.95,30.48 | 107.95,30.48 113.67,30.48 | 113.67,30.48 119.38,30.48 | 119.38,30.48 125.09,30.48 | 125.09,30.48 130.81,30.48 | 130.81,30.48 136.53,30.48 | 136.53,30.48 141.6,30.48 142.24,29.84 142.24,28.69 R8.A | R7.A 136.64,30.36 136.53,30.48 | R6.A 130.93,30.36 130.81,30.48 | R5.A 125.21,30.36 125.09,30.48 | R4.A 119.5,30.36 119.38,30.48 | R3.A 113.78,30.36 113.67,30.48 | R2.A 108.06,30.36 107.95,30.48 | U$5.O2 21.84,22.29 22.23,21.91
  Top 0.406: U$18.A1 U$18.A2 U$18.A3 U$3.A2 | IC2.18 70.36,23.62 69.85,24.13 69.85,27.58 CB3.2 CA3.2 65.38,26.01 v64.77,25.4 | 62.71,17.14 IC2.6 | 28.89,22.54 28.89,30.16 29.84,31.11 54.61,31.11 55.24,30.48 v55.24,26.67
  Top 0.61: 69.22,28.22 CB3.2
  Top 0.813: IC2.18 73.15,23.62 73.66,24.13 73.66,24.77 74.3,25.4 88.9,25.4 93.34,29.84 97.16,29.84 | 97.16,29.84 102.23,29.84 102.35,29.96 | C1.+ 96.77,29.46 97.16,29.84
  Bottom 0.406: v64.77,25.4 56.52,25.4 v55.24,26.67
  Bottom 0.813: U$3.B2 U$3.A2
REG_5V_BUS  (via drill 0.5)
  Top 0.305: RNB.5 31.66,20.87 v31.75,20.95
  Top 0.61: X1.3 37.34,12.38 | X3.2 53.98,12.06
  Bottom 0.406: 37.34,12.38 X1.3 | 53.98,12.06 X3.2
  Bottom 0.813: 37.34,12.38 37.34,11.05 39.37,8.89 52.7,8.89 53.98,10.16 53.98,12.06
  Bottom 1.016: 37.34,12.38 34.86,10.16 33.34,10.16 31.75,11.75 v31.75,20.95
REG_5V_EXT  (via drill 0.5, 0.6)
  Top 0.406: U$5.O1 v17.14,24.13
  Top 0.813: CB2.2 CA2.2 9.76,15.64 8.89,16.51 | 8.89,16.51 IC1.1 | v10.92,17.91 10.92,17.27 10.16,16.51 8.89,16.51
  Bottom 0.813: v17.14,24.13 v10.92,17.91
UNREG_12V  (via drill 0.5, 0.9)
  Top 0.762: v95.38,13.46 IC3.10
  Top 1.524: v43.18,29.21 43.18,24.13 41.91,22.86 36.7,22.86 32.89,19.05 32.89,9.08 29.11,5.3 28.57,4.76
  Top 1.676: v43.18,29.21 40.51,29.21 C2.+
  Top 2.286: BRA1.~@2 22.86,14.61 16.01,14.61
  Top 2.54: 16.01,14.61 U$1.TIP | X2.2 28.55,4.45 28.57,4.76 | BRA1.~@2 BRA1.~@1 24.13,12.45 28.57,8 28.57,5.84 29.11,5.3
  Bottom 1.27: 98.81,33.02 98.81,16.89 v95.38,13.46
  Bottom 1.676: K2.2 160.66,57.78 163.19,55.24 163.19,46.35 K1.2 160.66,38.73 158.12,36.2 120.02,36.2 | K4.2 124.46,57.78 127,55.24 127,46.35 K3.2 124.46,40.64 120.02,36.2 | K6.2 75.56,57.78 78.11,55.24 78.11,46.35 K5.2 75.56,37.47 71.12,33.02 | K8.2 38.73,57.78 41.27,55.24 41.27,46.35 K7.2 38.73,37.47 43.18,33.02 | 120.02,36.2 101.6,36.2 98.42,33.02
  Bottom 1.778: v43.18,29.21 43.18,33.02 71.12,33.02 98.42,33.02 98.81,33.02

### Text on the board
tNames: Bank 1 | 8 | 6 | 4 | 2 | 7 | 5 | 3 | 1 | Address | A0 | A1 | A2 | PULL-UP | I2C 5V | I2C IN | I2C OUT | GND | +5V | SDA | SCL | SCL | SDA | +5V | +5V | GND | MCP23008 | I2CR8x0 | REV.A | 2016 ControlEverything.com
